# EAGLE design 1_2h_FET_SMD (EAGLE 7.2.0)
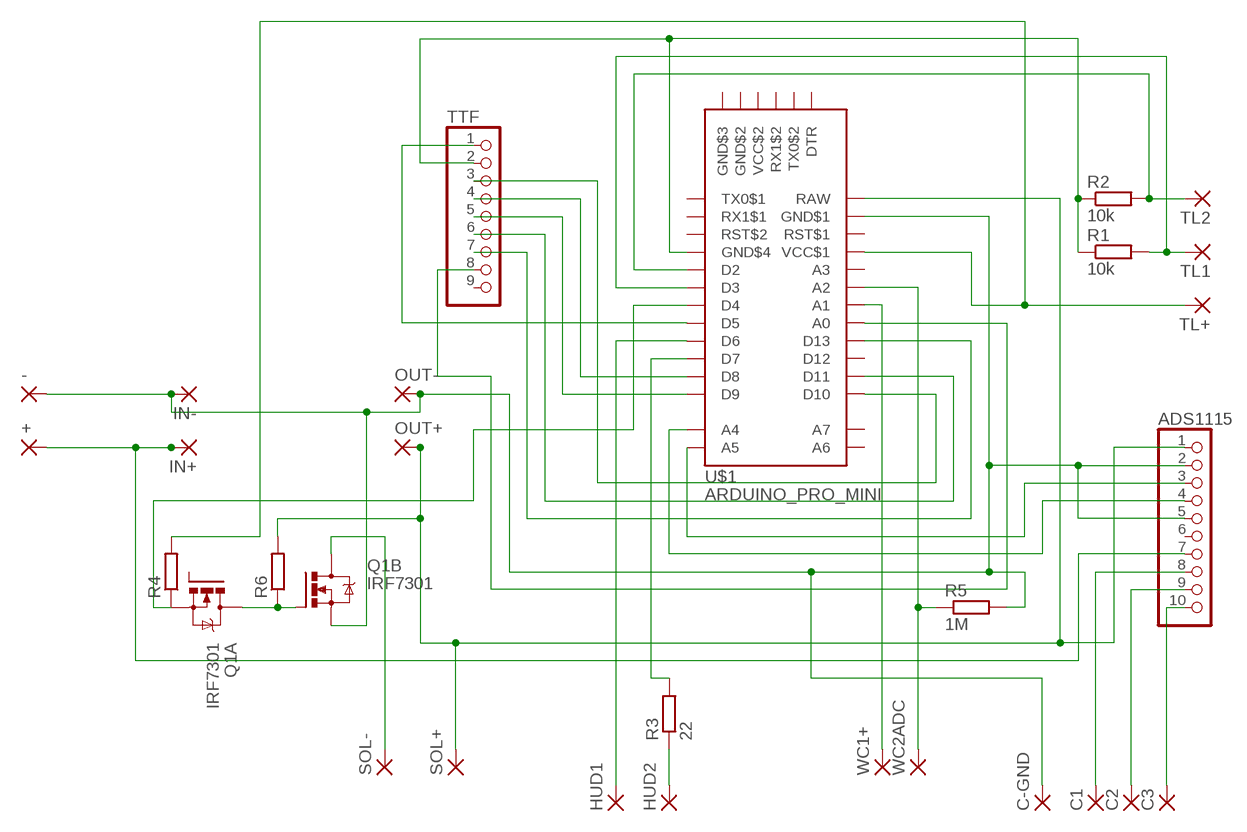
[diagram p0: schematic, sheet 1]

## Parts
+  2,54/1,0  [2,54/1,0]
-  2,54/1,0  [2,54/1,0]
ADS1115  PINHD-1X10  [1X10]
C1  2,54/1,1  [2,54/1,1]
C2  2,54/1,1  [2,54/1,1]
C3  2,54/1,1  [2,54/1,1]
C-GND  2,54/1,1  [2,54/1,1]
HUD1  2,54/1,0  [2,54/1,0]
HUD2  2,54/1,0  [2,54/1,0]
IN+  1,6/0,8  [1,6/0,8]
IN-  1,6/0,8  [1,6/0,8]
OUT+  1,6/0,8  [1,6/0,8]
OUT-  1,6/0,8  [1,6/0,8]
Q1  IRF7301  FDS6890A  [M08A]
R1  10k  R-EU_0204/5  [0204/5]
R2  10k  R-EU_0204/5  [0204/5]
R3  22  R-EU_0204/5  [0204/5]
R4  R-EU_R1210W  [R1210W]
R5  1M  R-EU_0204/5  [0204/5]
R6  R-EU_R1210W  [R1210W]
SOL+  2,54/1,0  [2,54/1,0]
SOL-  2,54/1,0  [2,54/1,0]
TL1  2,54/1,0  [2,54/1,0]
TL2  2,54/1,0  [2,54/1,0]
TL+  2,54/1,0  [2,54/1,0]
TTF  PINHD-1X9  [1X09]
U$1  ARDUINO_PRO_MINI  [ARDUINO_PRO_MINI]
WC1+  2,54/1,0  [2,54/1,0]
WC2ADC  2,54/1,0  [2,54/1,0]

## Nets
+5V: ADS1115.1 OUT+.1(P) R6.2 SOL+.1(P) U$1.RAW
GND: -.1(P) ADS1115.2 ADS1115.5 C-GND.1(P) IN-.1(P) OUT-.1(P) Q1.3(B:S) R5.2 U$1.GDN$1(GND$1)
N$3: R4.2 TL+.1(P) U$1.VCC$1
N$4: R2.2 TL2.1(P) U$1.D2
N$5: R1.2 TL1.1(P) U$1.D3
N$6: TTF.3 U$1.D10
N$7: TTF.4 U$1.D8
N$8: TTF.5 U$1.D9
N$9: TTF.6 U$1.D11
N$10: TTF.7 U$1.D13
N$11: TTF.8 U$1.A0
N$12: TTF.1 U$1.D5
N$13: ADS1115.3 U$1.A5
N$14: ADS1115.4 U$1.A4
N$15: +.1(P) ADS1115.7 IN+.1(P)
N$16: HUD1.1(P) U$1.D6
N$17: HUD2.1(P) R3.1
N$18: R3.2 U$1.D7
N$19: R1.1 R2.1 TTF.2 U$1.GND$4
N$20: Q1.1(A:S) R4.1 U$1.D4
N$21: Q1.5(B:D) Q1.6(B:D) SOL-.1(P)
N$22: U$1.A1 WC1+.1(P)
N$23: R5.1 U$1.A2 WC2ADC.1(P)
N$29: ADS1115.10 C3.1(P)
N$31: ADS1115.9 C2.1(P)
N$36: ADS1115.8 C1.1(P)
N$39: Q1.4(B:G) Q1.7(A:D) Q1.8(A:D) R6.1
Unconnected: ADS1115.6 Q1.2(A:G) TTF.9 U$1.A3 U$1.A6 U$1.A7 U$1.D12 U$1.DTR U$1.RST$1 U$1.RST$2 U$1.RX1$1 U$1.RX1$2 U$1.TX0$1 U$1.TX0$2

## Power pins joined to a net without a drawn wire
GND$2: U$1.GND$2
GND$3: U$1.GND$3
VCC$2: U$1.VCC$2

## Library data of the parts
+ - HUD1 HUD2 SOL+ SOL- TL1 TL2 TL+ WC1+ WC2ADC = wirepad:2,54/1,0: THROUGH-HOLE PAD
ADS1115 = pinhead:PINHD-1X10: PIN HEADER
C1-C3 C-GND = wirepad:2,54/1,1: THROUGH-HOLE PAD
IN+ IN- OUT+ OUT- = wirepad:1,6/0,8: THROUGH-HOLE PAD
Q1 = transistor-power:FDS6890A: Dual N-Channel 2.5V Specified PowerTrenchTM MOSFET Source: FDS6890A.pdf
R1-R6 = resistor:R-EU_: RESISTOR, European symbol
TTF = pinhead:PINHD-1X9: PIN HEADER
U$1 = srg:ARDUINO_PRO_MINI: Arduino Pro-Mini Made by Sparkfun Comes in 3.3 volt and 5 volt versions Note: A6 & A7 are analog in only

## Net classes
0 default: clearance 0.205 mm

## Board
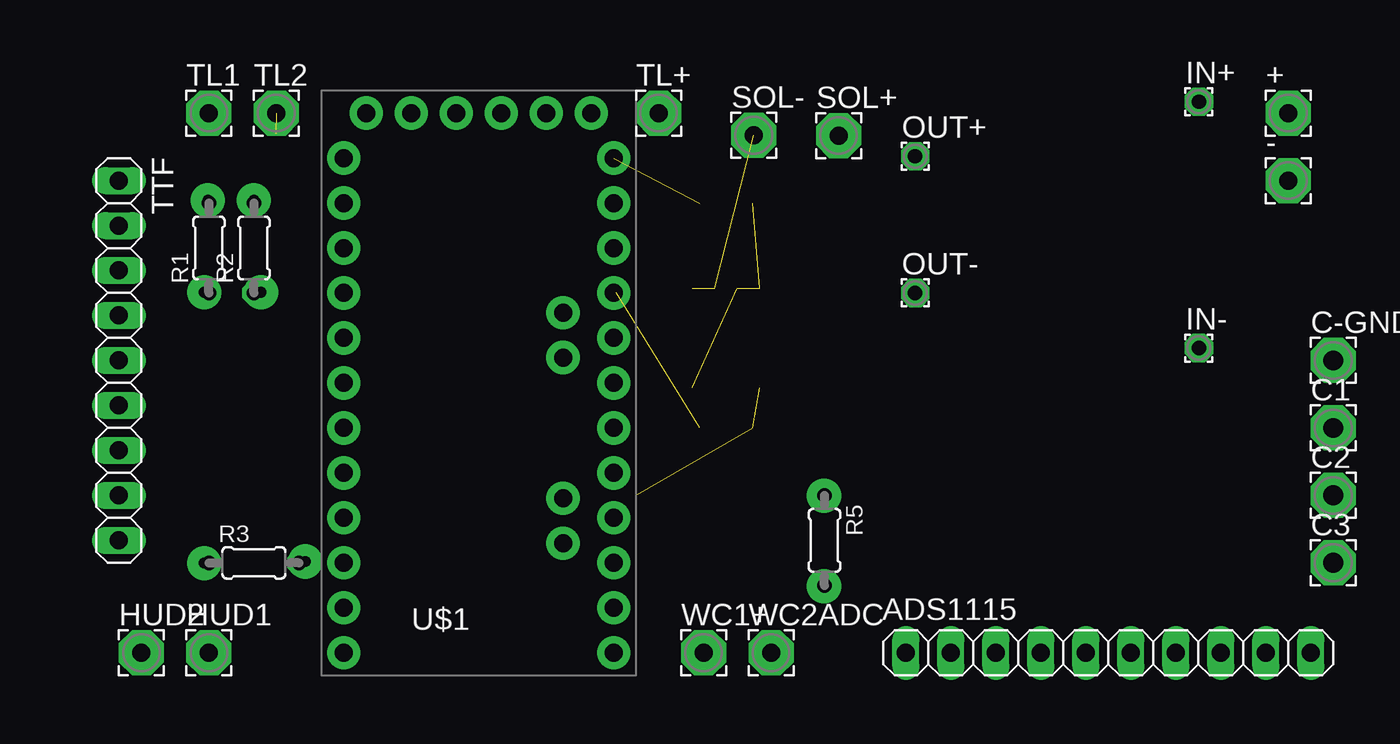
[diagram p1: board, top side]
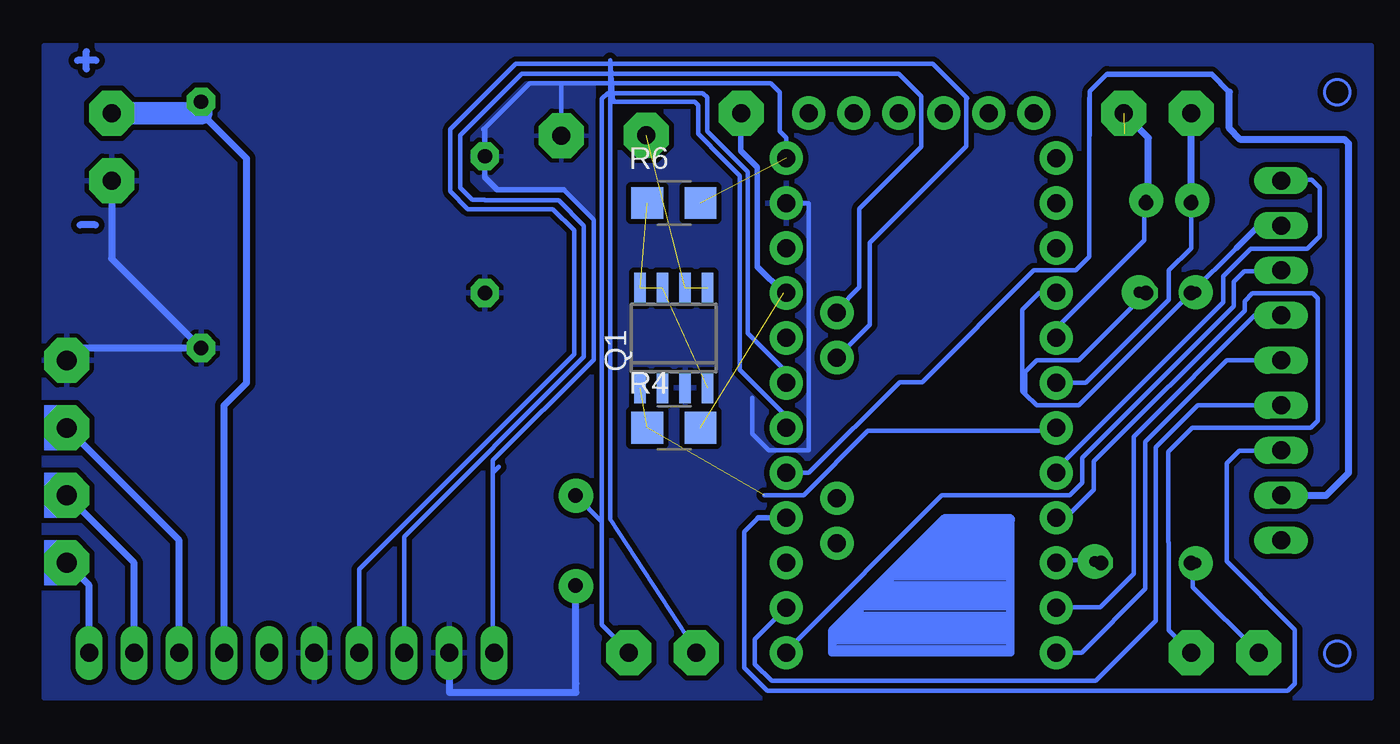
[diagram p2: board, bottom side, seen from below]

No outline drawn. Coordinates in mm, seen from the top.
Copper layers (1*16): Top 0.035mm / dielectric 1.5mm / Bottom 0.035mm
Design rules "1_2b": minimum track width 10mil, minimum drill 24mil, track to track 0.205mm, track to pad 0.205mm, pad to pad 0.205mm, via to via 0.205mm, smd to smd 8mil, copper to edge 40mil, drill to drill 8mil, minimum pad ring 10mil, minimum via ring 8mil, stop-mask expansion 4mil, vias tented up to drill 0mil, thermal gap 10mil

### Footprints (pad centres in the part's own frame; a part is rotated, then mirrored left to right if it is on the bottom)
2,54/1,0 = drill 1.016 pad 2.54 octagon: 1 0,0
1X10 = drill 1.016 long: 1 -11.43,0; 2 -8.89,0; 3 -6.35,0; 4 -3.81,0; 5 -1.27,0; 6 1.27,0; 7 3.81,0; 8 6.35,0; 9 8.89,0; 10 11.43,0
2,54/1,1 = drill 1.118 pad 2.54 octagon: 1 0,0
1,6/0,8 = drill 0.813 pad 1.6 octagon: 1 0,0
M08A = smd 0.65 x 1.75: 1 -1.905,-2.8; 2 -0.635,-2.8; 3 0.635,-2.8; 4 1.905,-2.8; 5 1.905,2.8; 6 0.635,2.8; 7 -0.635,2.8; 8 -1.905,2.8
0204/5 = drill 0.813 octagon: 1 -2.54,0; 2 2.54,0
R1210W = smd 1.8 x 1.8: 1 -1.499,0; 2 1.499,0
1X09 = drill 1.016 long: 1 -10.16,0; 2 -7.62,0; 3 -5.08,0; 4 -2.54,0; 5 0,0; 6 2.54,0; 7 5.08,0; 8 7.62,0; 9 10.16,0
ARDUINO_PRO_MINI = drill 1.016 pad 1.88: A0 7.62,-5.08; A1 7.62,-2.54; A2 7.62,0; A3 7.62,2.54; A4 4.763,1.429; A5 4.763,3.969; A6 4.763,-9.049; A7 4.763,-6.509; D2 -7.62,2.54; D3 -7.62,0; D4 -7.62,-2.54; D5 -7.62,-5.08; D6 -7.62,-7.62; D7 -7.62,-10.16; D8 -7.62,-12.7; D9 -7.62,-15.24; D10 7.62,-15.24; D11 7.62,-12.7; D12 7.62,-10.16; D13 7.62,-7.62; DTR 6.35,15.24; GDN$1 7.62,10.16; GND$2 -3.81,15.24; GND$3 -6.35,15.24; GND$4 -7.62,5.08; RAW 7.62,12.7; RST$1 7.62,7.62; RST$2 -7.62,7.62; RX1$1 -7.62,10.16; RX1$2 1.27,15.24; TX0$1 -7.62,12.7; TX0$2 3.81,15.24; VCC$1 7.62,5.08; VCC$2 -1.27,15.24

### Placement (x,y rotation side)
+  71.12,33.02 0 top
-  71.12,29.21 0 top
ADS1115  60.96,2.54 0 top
C1  73.66,15.24 0 top
C2  73.66,11.43 0 top
C3  73.66,7.62 0 top
C-GND  73.66,19.05 0 top
HUD1  10.16,2.54 0 top
HUD2  6.35,2.54 0 top
IN+  66.07,33.66 0 top
IN-  66.07,19.75 0 top
OUT+  50.05,30.58 0 top
OUT-  50.05,22.86 0 top
Q1  39.37,20.32 0 bottom
R1  10.16,25.4 90 top
R2  12.7,25.4 90 top
R3  12.7,7.62 0 top
R4  39.37,15.24 0 bottom
R5  44.93,8.89 270 top
R6  39.37,27.94 0 bottom
SOL+  45.72,31.75 0 top
SOL-  40.94,31.77 0 top
TL1  10.16,33.02 0 top
TL2  13.97,33.02 0 top
TL+  35.56,33.02 0 top
TTF  5.08,19.05 270 top
U$1  25.4,17.78 0 top
WC1+  38.1,2.54 0 top
WC2ADC  41.91,2.54 0 top

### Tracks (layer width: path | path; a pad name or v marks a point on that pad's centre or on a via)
+5V  (1 unrouted)
  Bottom 0.254: U$1.RAW 33.02,31.62 33.4,32 33.4,34.2 33.9,34.7 45.72,34.7 | 45.72,34.7 47.5,34.7 50.1,32.1 | 45.6,28.7 43.9,27 43.9,19.1 49.6,13.4 49.6,12.7 | 49.6,12.7 49.6,2.61 ADS1115.1 | SOL+.1 45.72,34.7 | 49.26,13.04 49.6,12.7
  Bottom 0.305: 50.1,32.1 50.05,32.1 OUT+.1 50.05,29.4 49.35,28.7 45.6,28.7
  pour Bottom: 43.9,27 45.6,28.7 50.25,28.7 50.75,29.2 50.75,31.65 47.7,34.7 43.9,34.7
GND
  Bottom 0.254: U$1.GDN$1 31.75,27.94 31.75,13.97 34.02,13.97 34.95,14.9 34.95,16.95
  Bottom 0.406: -.1 71.12,24.8 IN-.1 72.96,19.75 C-GND.1 | ADS1115.2 52.05,2.54 52.05,0.3 44.9,0.3 44.9,0.8 44.93,0.8 R5.2
  pour Bottom (isolate 0.3): 0,36.83 74.93,36.83 74.93,0 0,0
N$1
  Bottom 0.406: 20.32,9.98 20.32,2.54 30.48,2.54 30.48,3.81 24.13,10.16 20.32,10.16 20.32,9.98 | 20.32,9.98 20.5,9.8 24.1,9.8 24.3,9.6 20.7,9.6 20.5,9.4 24.4,9.4 24.6,9.2 20.7,9.2 20.5,9 24.8,9 25,8.8 20.7,8.8 20.4,8.5 25.1,8.5 25.2,8.6 25.5,8.3 20.6,8.3 20.4,8.1 25.7,8.1 26,7.8 20.6,7.8 20.4,7.6 26.2,7.6 26.5,7.3 20.5,7.3 20.4,7.2 26.6,7.2 26.9,6.9 20.5,6.9 20.4,6.8 27,6.8 27.4,6.4 20.6,6.4 20.4,6.2 27.6,6.2 27.9,5.9 20.6,5.9 20.4,5.7 28.2,5.7 28.5,5.4 20.7,5.4 20.4,5.1 28.7,5.1 | 28.7,5.1 28.9,4.9 | 28.9,4.9 28.9,5 28.7,5.2 28.7,5.1 | 28.9,4.9 29.1,4.7 20.4,4.7 20.4,4.5 20.5,4.4 29.2,4.4 29.3,4.5 29.7,4.1 | 29.7,4.1 30,4.1 | 29.7,4.1 20.5,4.1 20.4,4 20.4,3.8 30.2,3.8 30.2,3.6 30.3,3.5 20.4,3.5 20.4,3.2 30.4,3.2 30.4,2.8 20.4,2.8 20.4,9.8 20.5,9.9 24,9.9 24.1,10 24.1,9.9 30.3,3.7
N$3  (1 unrouted)
  Bottom 0.305: U$1.VCC$1 33.16,22.86 34.65,24.35 34.65,29.95 35.6,30.9 35.6,32.98 TL+.1
N$4  (1 unrouted)
  Bottom 0.178: 13.95,31.86 13.97,31.86
  Bottom 0.254: 12.57,28.12 R2.2 12.8,27.89 12.8,25.83 17.6,21.03 17.6,20.34 U$1.D2
  Bottom 0.406: 12.57,28.12 12.57,31.62 TL2.1
N$5
  Bottom 0.254: R1.2 10.16,25.4 11.43,24.13 11.43,22.47 16.1,17.8 17.76,17.8 U$1.D3
  Bottom 0.406: R1.2 TL1.1
N$6
  Bottom 0.254: U$1.D10 32.92,2.74 24.23,11.43 17.02,11.43 16.3,12.15 16.3,13.55 7.75,22.1 7.75,23.5 7.15,24.1 5.11,24.1 TTF.3
N$7
  Bottom 0.254: TTF.4 6.56,21.59 13.4,14.75 13.4,7 15.3,5.1 17.76,5.1 U$1.D8
N$8
  Bottom 0.254: 17.6,2.74 U$1.D9 16.35,2.55 12.75,6.15 12.75,14.45 8.15,19.05 TTF.5
N$9
  Bottom 0.254: U$1.D11 34.8,3.3 34.8,1.9 33.85,0.95 15.56,0.95 12.15,4.36 12.15,14.15 9.79,16.51 TTF.6
N$10
  Bottom 0.254: 34.61,10.16 35.4,9.37 35.4,1.7 34.1,0.4 4.7,0.4 4.32,0.78 4.3,0.78 4.3,3.85 8.15,7.7 8.15,13.25 7.45,13.95 5.1,13.95 TTF.7
  Bottom 0.305: 34.61,10.16 U$1.D13
N$11
  Bottom 0.178: 14.86,35.2
  Bottom 0.254: 14.86,35.2 14.9,35.24 15.88,34.27 15.88,33.9 | 15.88,31.75 15.88,33.9 | 15.88,33.9 15.9,33.88 15.9,24.9 16.67,24.13 19.05,24.13 25.35,17.83 26.62,17.83 31.75,12.7 U$1.A0
  Bottom 0.305: 14.86,35.2 9,35.2 8,34.2 | 1.27,13.97 1.27,31.3
  Bottom 0.406: TTF.8 2.54,11.43 1.27,12.7 1.27,31.3 1.5,31.52 7.38,31.52 8,32.15 8,34.2
N$12
  Bottom 0.254: TTF.1 5.04,29.25 3.35,29.25 2.9,28.8 2.9,26.05 3.6,25.35 6.8,25.35 8.35,23.8 8.35,22.35 17.25,13.45 17.25,13.23 U$1.D5
N$13
  Bottom 0.254: 54.41,2.74 ADS1115.3 54.6,9.1 44.45,19.25 44.45,26.67 45.88,28.1 50.04,28.1 50.06,28.12 50.75,28.12 51.44,28.8 51.44,31.77 47.97,35.24 26.67,35.24 25.4,33.97 25.4,31.11 28.89,27.62 28.89,23.18 30.12,21.95 30.18,21.95 U$1.A5
N$14
  Bottom 0.254: ADS1115.4 57.15,7.25 45,19.4 45,26.4 46.2,27.6 51,27.6 52,28.6 52,32.1 48.3,35.8 24.75,35.8 22.8,33.85 22.85,33.8 22.85,31.15 28.3,25.7 28.3,21.07 U$1.A4
N$15
  Bottom 0.406: ADS1115.7 64.77,16.51 63.5,17.78 63.5,30.45 66.07,33.02
  Bottom 1.27: +.1 66.07,33.02 IN+.1
N$16
  Bottom 0.254: U$1.D6 17.25,10.16 15.65,11.76 15.65,13.35 7.14,21.86 7.14,22.41 6.7,22.85 3.3,22.85 3,22.55 3,15.65 3.4,15.25 10.1,15.25 11.45,13.9 11.45,8.79 11.43,8.77 11.43,3.81 HUD1.1
N$17
  Bottom 0.254: 10.06,7.54 R3.1 | 10.06,7.52 10.06,6.25 HUD2.1
  Bottom 0.305: 10.06,7.54 10.06,7.52
N$18
  Bottom 0.254: R3.2 15.32,7.77 17.6,7.77 U$1.D7
N$19
  Bottom 0.254: 7.62,25.4 R1.1 16.51,16.51 18.89,16.51 19.53,17.14 | 19.53,17.14 19.53,18.41 18.89,19.05 16.51,19.05 R2.1 | U$1.GND$4 18.73,22.86 19.68,21.91 19.68,17.3 19.53,17.14
  Bottom 0.305: TTF.2 6.35,26.67 7.62,25.4
N$20  (2 unrouted)
  Bottom 0.254: U$1.D4 17.83,15.09 28.41,15.09 32.05,11.45 34.27,11.45
N$21  (2 unrouted)
N$22
  Bottom 0.254: U$1.A1 33.15,15.32 33.15,16 35.66,18.52 35.66,29.49 36.58,30.4 36.58,30.43 38,31.85 38,33.45 38.2,33.65 42.8,33.65 42.98,36.02 42.98,10.08 38.18,2.74 WC1+.1
N$23
  Bottom 0.254: 43.43,9.94 43.43,33.82 43.1,34.15 37.75,34.15 37.5,33.9 37.5,32 36.36,30.86 36.35,30.86 35.2,29.72 35.2,20.57 33.15,18.52 33.15,17.83 U$1.A2 | WC2ADC.1 42.06,2.74 43.43,4.12 43.43,9.94 | 43.43,9.94 R5.1
N$28
  Bottom 0.406: 72.55,35.5 72.55,36.5
N$29
  Bottom 0.406: ADS1115.10 72.39,6.35 C3.1
N$30
  Bottom 0.178: 72,36 73,36
  Bottom 0.406: 72,36 73.05,36
N$31
  Bottom 0.406: ADS1115.9 69.85,7.62 C2.1
N$32
  Bottom 0.178: 72.5,35.5 72.5,36.4
N$33
  Bottom 0.178: 72,26.7 72.05,26.7
  Bottom 0.406: 72.05,26.7 72.9,26.7
N$34  (via drill 0.6 pad 1.93)
  other vias: 44.9,11.4
N$35  (via drill 0.6 pad 1.93)
  other vias: 44.9,6.3
N$36
  Bottom 0.406: ADS1115.8 67.31,8.89 C1.1
N$37  (via drill 0.6 pad 1.93)
  other vias: 12.7,28.1
N$38  (via drill 0.6 pad 1.93)
  other vias: 10.1,28.1
N$39  (3 unrouted)
N$40  (via drill 0.6 pad 1.93)
  other vias: 9.9,7.6
N$41  (via drill 0.6 pad 1.93)
  other vias: 15.6,7.7
N$42  (via drill 0.6 pad 1.93)
  other vias: 9.9,22.9
N$43  (via drill 0.6 pad 1.93)
  other vias: 13.1,22.9
(copper drawn outside any net)
  shapes: Bottom area x4, Bottom circle x2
